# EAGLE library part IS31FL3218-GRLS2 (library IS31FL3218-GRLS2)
IC LED DRIVER 18CH CC PWM 24SOIC Source: Datasheet
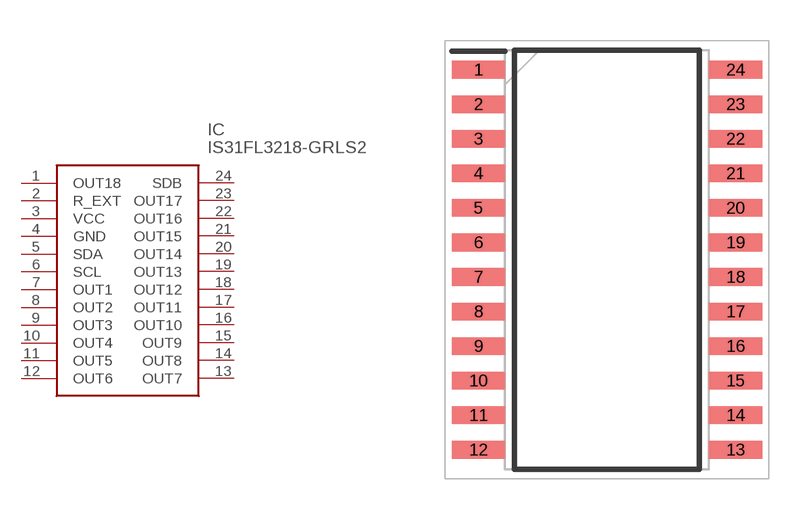
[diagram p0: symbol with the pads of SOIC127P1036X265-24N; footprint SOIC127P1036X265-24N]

Designator prefix IC

## IS31FL3218-GRLS2 (Description: IC LED DRIVER 18CH CC PWM 24SOIC; Height: 2.65mm; Manufacturer_Name: Lumissil; Manufacturer_Part_Number: IS31FL3218-GRLS2; Mouser_Part_Number: 870-IS31FL3218-GRLS2; Mouser_Price-Stock: https://www.mouser.co.uk/ProductDetail/Lumissil/IS31FL3218-GRLS2?qs=iHGOLYL7GwC17lH0po6WyQ%3D%3D)  [SOIC127P1036X265-24N]
1  OUT18
2  R_EXT
3  VCC
4  GND
5  SDA
6  SCL
7  OUT1
8  OUT2
9  OUT3
10  OUT4
11  OUT5
12  OUT6
13  OUT7
14  OUT8
15  OUT9
16  OUT10
17  OUT11
18  OUT12
19  OUT13
20  OUT14
21  OUT15
22  OUT16
23  OUT17
24  SDB

## Footprint SOIC127P1036X265-24N (pad centres in mm)
SOP-24
smd 1.95 x 0.65: 1 -4.725,6.985; 2 -4.725,5.715; 3 -4.725,4.445; 4 -4.725,3.175; 5 -4.725,1.905; 6 -4.725,0.635; 7 -4.725,-0.635; 8 -4.725,-1.905; 9 -4.725,-3.175; 10 -4.725,-4.445; 11 -4.725,-5.715; 12 -4.725,-6.985; 13 4.725,-6.985; 14 4.725,-5.715; 15 4.725,-4.445; 16 4.725,-3.175; 17 4.725,-1.905; 18 4.725,-0.635; 19 4.725,0.635; 20 4.725,1.905; 21 4.725,3.175; 22 4.725,4.445; 23 4.725,5.715; 24 4.725,6.985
